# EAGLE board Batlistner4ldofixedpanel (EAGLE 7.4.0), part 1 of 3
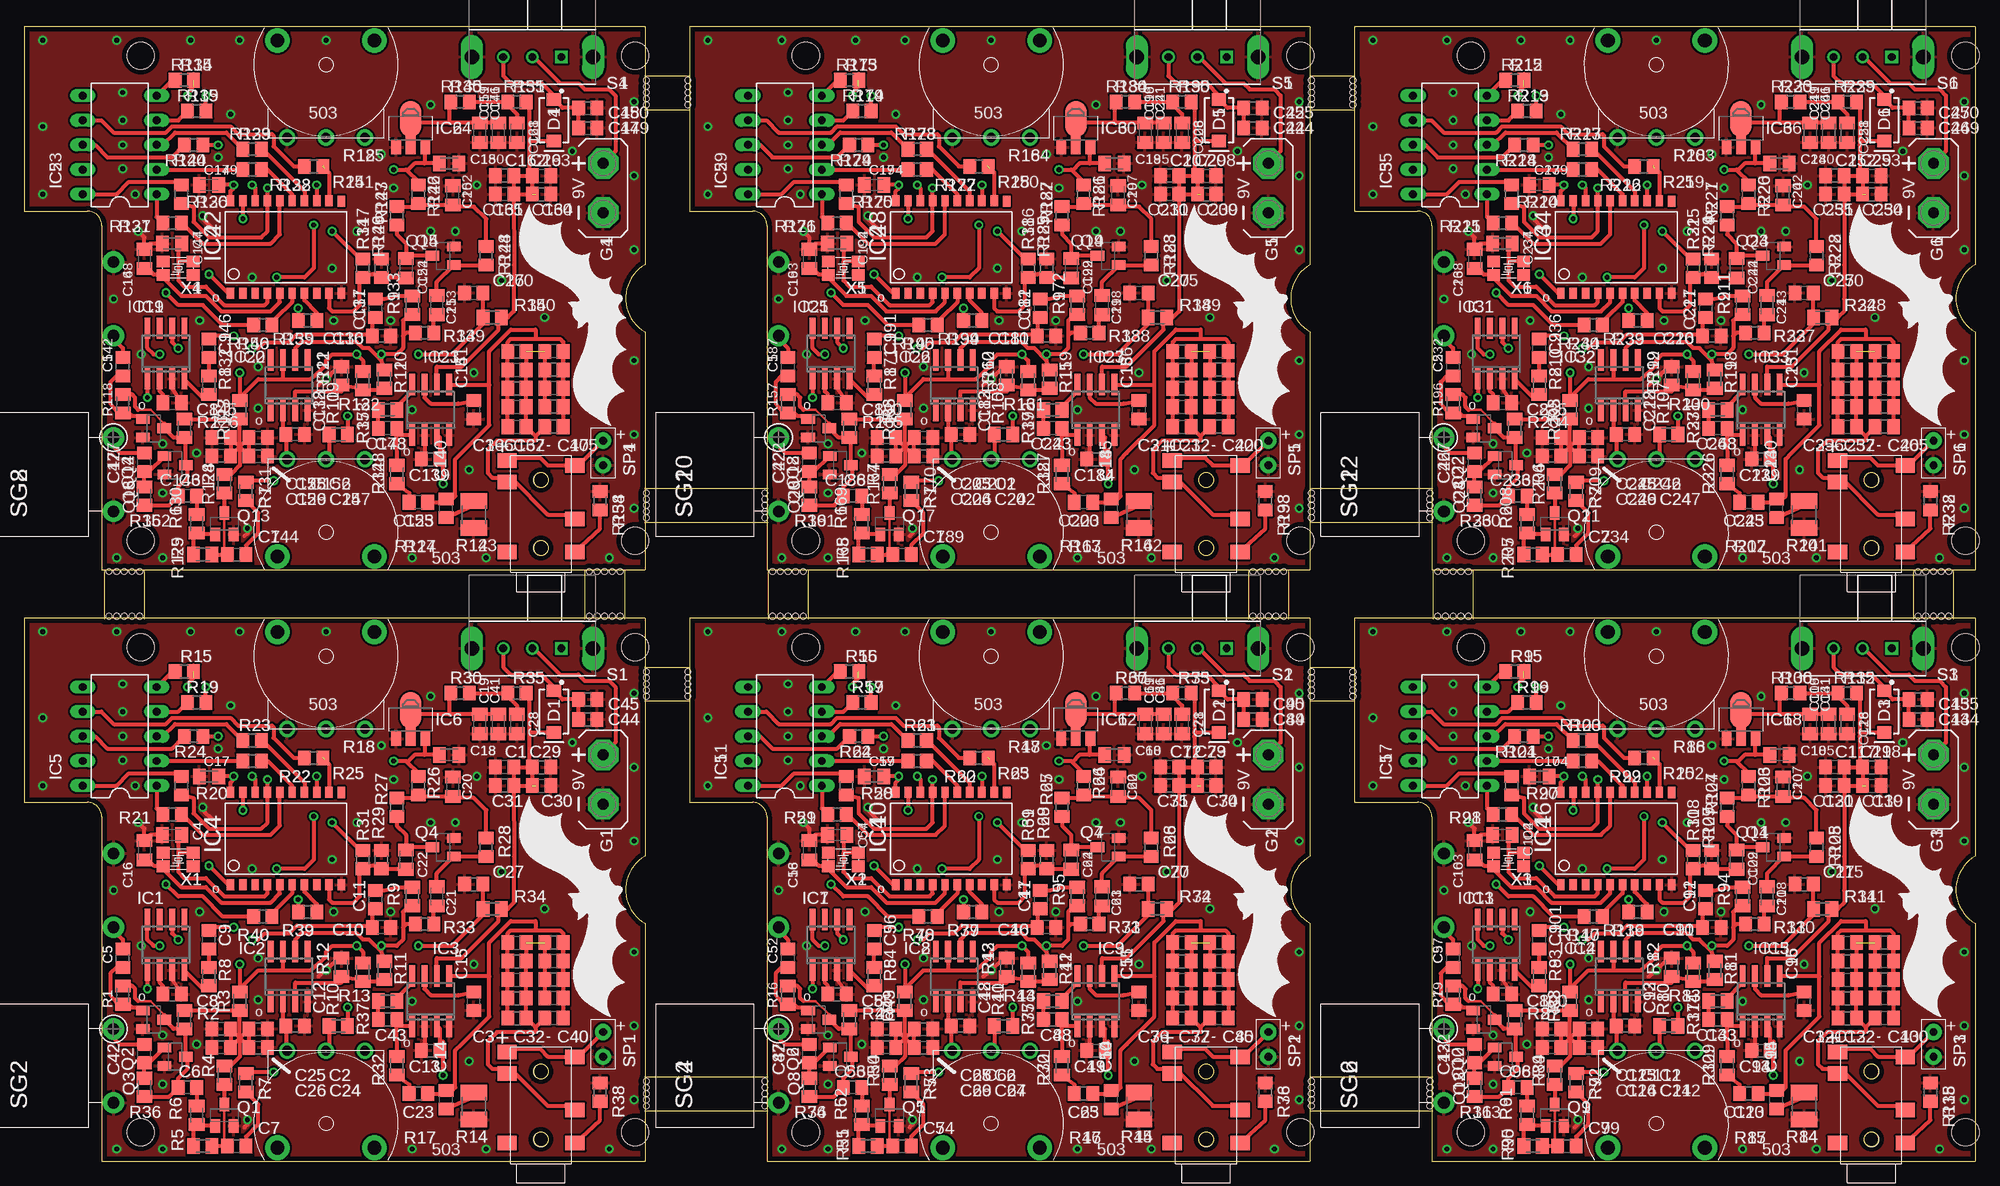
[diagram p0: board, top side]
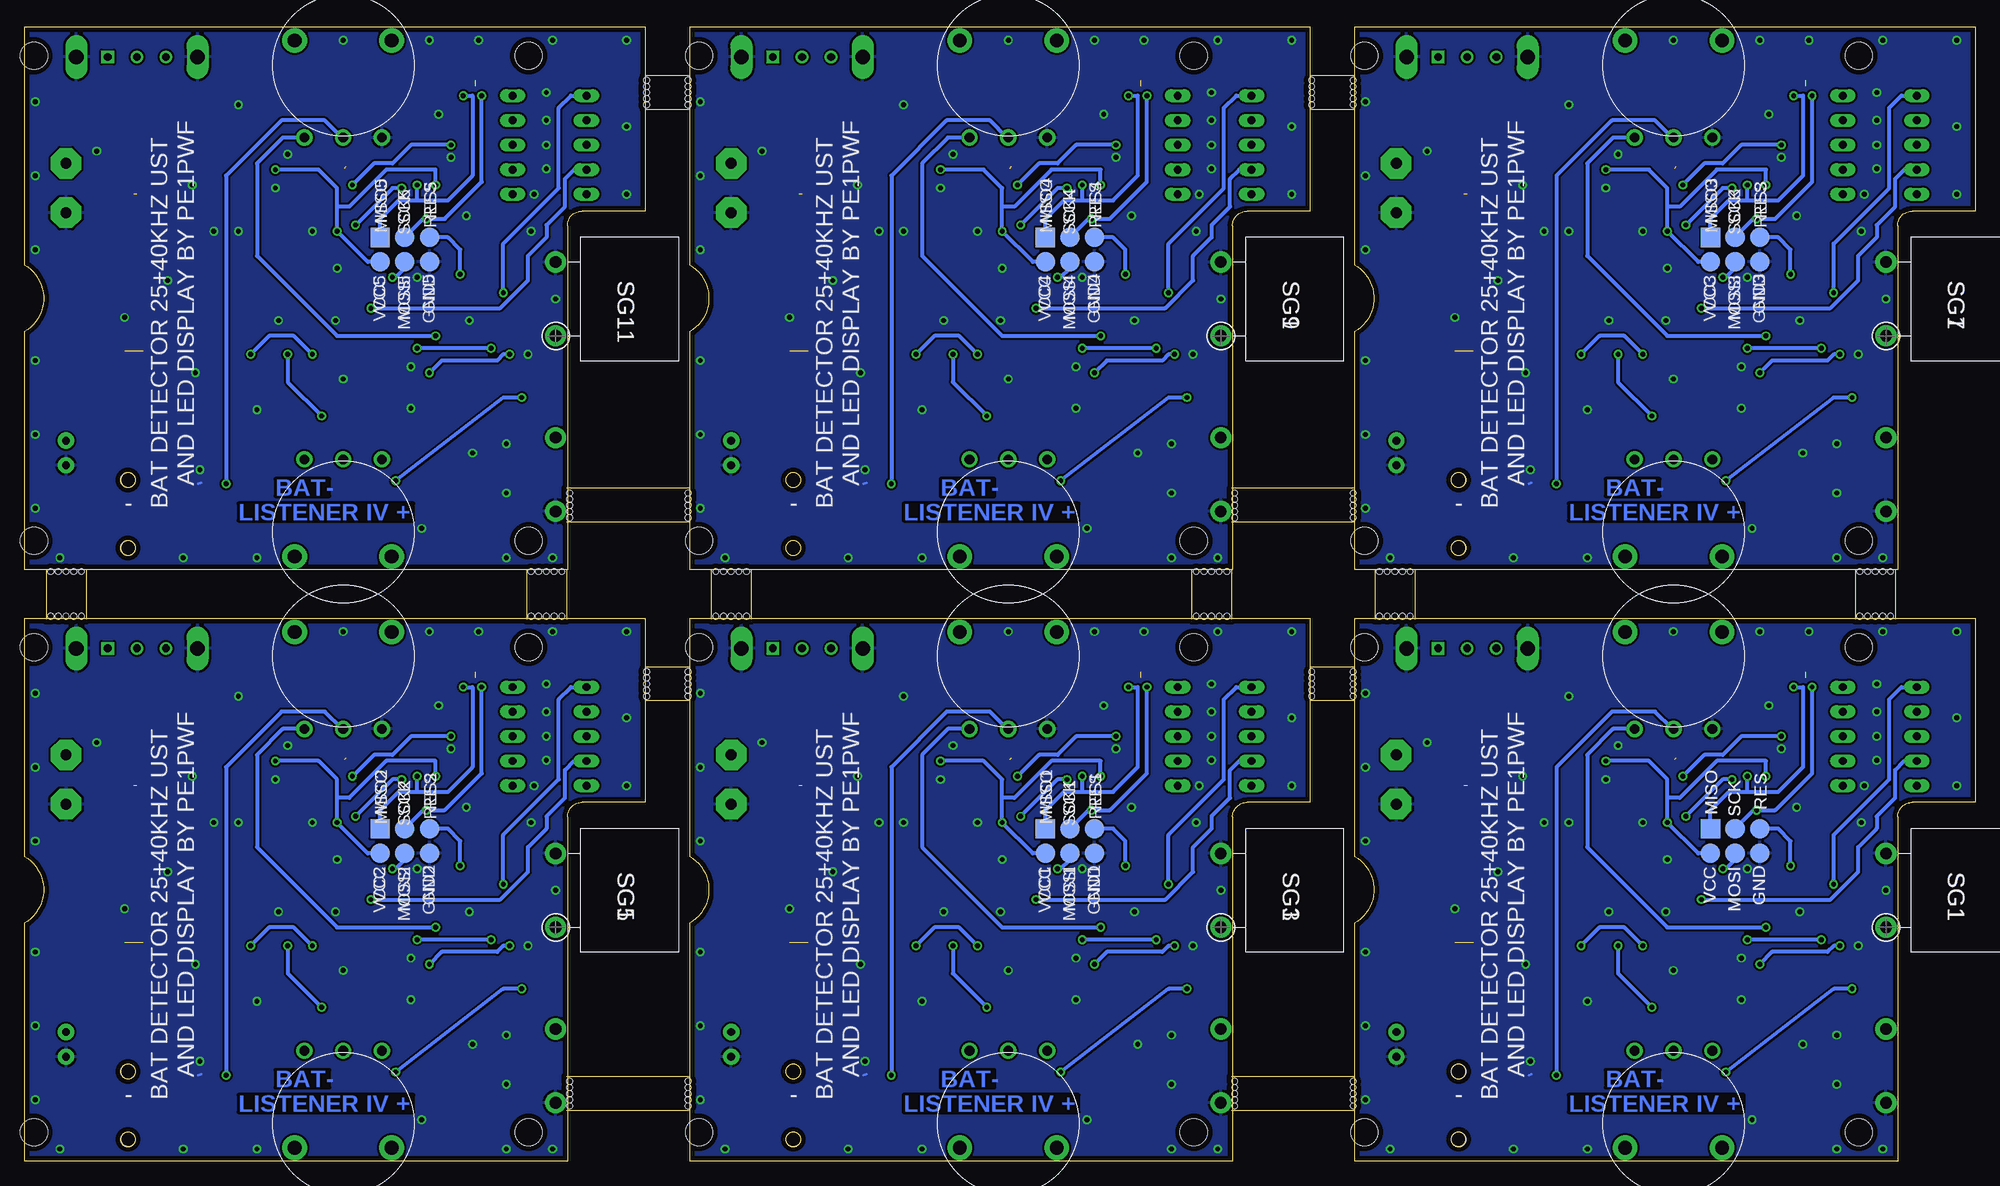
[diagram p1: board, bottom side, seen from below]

Size 201.16 x 116.96 mm. Coordinates in mm from the lower left corner, seen from the top.
Outline: 89 segments
Copper layers (1*16): Top 0.035mm / dielectric 1.5mm / Bottom 0.035mm
Design rules "default *": minimum track width 10mil, minimum drill 19mil, track to track 8mil, track to pad 8mil, pad to pad 8mil, via to via 8mil, smd to smd 8mil, copper to edge 20mil, drill to drill 8mil, minimum pad ring 10mil, minimum via ring 8mil, stop-mask expansion 4mil, vias tented up to drill 20mil, thermal gap 10mil
Holes 2.8 mm at 63,3 63,53 12,53 12,3 131.58,3 131.58,53 80.58,53 80.58,3 200.16,3 200.16,53 149.16,53 149.16,3 63,63.96 63,113.96 12,113.96 12,63.96 131.58,63.96 131.58,113.96 80.58,113.96 80.58,63.96 200.16,63.96 200.16,113.96 149.16,113.96 149.16,63.96
Holes 0.6 mm at 8.73,60.8 9.53,60.8 10.32,60.8 11.11,60.8 11.91,60.8 8.73,56.2 9.53,56.2 10.32,56.2 11.11,56.2 11.91,56.2 58.26,60.8 59.05,60.8 59.85,60.8 60.64,60.8 61.44,60.8 58.26,56.2 59.05,56.2 59.85,56.2 60.64,56.2 61.44,56.2 145.73,60.8 146.53,60.8 147.32,60.8 148.11,60.8 148.91,60.8 145.73,56.2 146.53,56.2 147.32,56.2 148.11,56.2 148.91,56.2 195.26,60.8 196.06,60.8 196.85,60.8 197.64,60.8 198.44,60.8 195.26,56.2 196.06,56.2 196.85,56.2 197.64,56.2 198.44,56.2 77.15,60.8 77.95,60.8 78.74,60.8 79.53,60.8 80.33,60.8 77.15,56.2 77.95,56.2 78.74,56.2 79.53,56.2 80.33,56.2 126.68,60.8 127.48,60.8 128.27,60.8 129.06,60.8 129.86,60.8 126.68,56.2 127.48,56.2 128.27,56.2 129.06,56.2 129.86,56.2 64.14,5.71 64.14,6.35 64.14,6.99 64.14,7.62 64.14,8.26 76.36,8.26 76.36,7.62 76.36,6.99 76.36,6.35 76.36,5.71 132.72,5.71 132.72,6.35 132.72,6.99 132.72,7.62 132.72,8.26 144.94,8.26 144.94,7.62 144.94,6.99 144.94,6.35 144.94,5.71 64.14,66.36 64.14,66.99 64.14,67.63 64.14,68.26 64.14,68.9 76.36,68.9 76.36,68.26 76.36,67.63 76.36,66.99 76.36,66.36 132.72,66.36 132.72,66.99 132.72,67.63 132.72,68.26 132.72,68.9 144.94,68.9 144.94,68.26 144.94,67.63 144.94,66.99 144.94,66.36 132.72,47.94 132.72,48.58 132.72,49.21 132.72,49.85 132.72,50.48 137,47.94 137,48.58 137,49.21 137,49.85 137,50.48 132.72,108.9 132.72,109.54 132.72,110.17 132.72,110.81 132.72,111.44 137,108.9 137,109.54 137,110.17 137,110.81 137,111.44 64.14,47.94 64.14,48.58 64.14,49.21 64.14,49.85 64.14,50.48 68.42,47.94 68.42,48.58 68.42,49.21 68.42,49.85 68.42,50.48 64.14,108.9 64.14,109.54 64.14,110.17 64.14,110.81 64.14,111.44 68.42,108.9 68.42,109.54 68.42,110.17 68.42,110.81 68.42,111.44

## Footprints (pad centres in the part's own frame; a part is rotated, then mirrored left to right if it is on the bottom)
C0805 = smd 1.3 x 1.5: 1 -0.95,0; 2 0.95,0
C0805K = smd 1.3 x 1.6: 1 -1,0; 2 1,0
SMA-DIODE = smd 1.27 x 1.47: A -2.15,0; C 2.15,0
AB9V = drill 1.118 pad 3.15 octagon: + 0,2.54; - 0,-2.54
TP20R = smd 2 x 2: TP 0,0
SO08 = smd 0.6 x 2.2: 1 -1.905,-2.6; 2 -0.635,-2.6; 3 0.635,-2.6; 4 1.905,-2.6; 5 1.905,2.6; 6 0.635,2.6; 7 -0.635,2.6; 8 -1.905,2.6
SO20L = smd 0.762 x 1.143: 1 -5.08,-5.131; 2 -3.81,-5.131; 3 -2.54,-5.131; 4 -1.27,-5.131; 5 0,-5.131; 6 1.27,-5.131; 7 2.54,-5.131; 8 3.81,-5.131; 9 5.08,-5.131; 10 6.35,-5.131; 11 6.35,4.369; 12 5.08,4.394; 13 3.81,4.394; 14 2.54,4.394; 15 1.27,4.394; 16 0,4.394; 17 -1.27,4.394; 18 -2.54,4.394; 19 -3.81,4.394; 20 -5.08,4.394
DIL10 = drill 0.813 long: 1 -5.08,-3.81; 2 -2.54,-3.81; 3 0,-3.81; 4 2.54,-3.81; 5 5.08,-3.81; 6 5.08,3.81; 7 2.54,3.81; 8 0,3.81; 9 -2.54,3.81; 10 -5.08,3.81
SOT89 = smd 1 x 1.5: 1 -1.499,-1.981; 3 1.499,-1.981 | smd 1 x 2: 2 0,-1.727 | smd 2.2 x 3.7: 2@1 0,0.94
TP20SQ = smd 2 x 2: TP 0,0
SOT23-BEC = smd 1 x 1.4: B -0.95,-1.1; C 0,1.1; E 0.95,-1.1
M0805 = smd 1.3 x 1.6: 1 -0.95,0; 2 0.95,0
R1210 = smd 1.6 x 2.7: 1 -1.4,0; 2 1.4,0
R0805 = smd 1.3 x 1.5: 1 -0.95,0; 2 0.95,0
RK10J11 = drill 1 pad 1.676: P$1 0,-7.5; P$2 -4,-7.5; P$3 4,-7.5 | drill 1.4 pad 2.54: P$4 5,2.5; P$5 -5,2.5
E-SWITCH_EG1206A_0 = drill 0.8 pad 1.3 square: 1 -3,3 | drill 0.8 pad 1.3: 2 0,3; 3 3,3 | drill 1.5 pad 1.778 long: 4 -6.25,3; 5 6.25,3
BMT1205XV7.5 = drill 1.2 pad 2.184: + 3.8,0; - -3.8,0
PADSONLY = drill 0.8 pad 1.676: + 0,0; - 0,-2.54
JW-PJ-342B = smd 1.5 x 2: P$1 4.1,1; P$2 4.1,8; P$3 7.5,1; P$4 11.3,8; P$5 13.5,8; P$6 13,1 | hole 1.5: 4.5,4.5; 11.5,4.5
IQG3225 = smd 1.3 x 1.2: 1 -1.55,-0.7; 2 1.55,-0.7; 3 1.55,0.7; 4 -1.55,0.7

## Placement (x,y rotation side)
C1  22uf  [C0805]  53.34,40.64 0 top
C2  22uf  [C0805]  24.13,13.65 0 top
C3  22uf  [C0805]  50.8,14.76 0 top
C4  22pF  [C0805K]  15.24,33.66 180 top
C5  1nF  [C0805]  10.16,20.95 90 top
C6  1nf  [C0805]  16.83,7.62 180 top
C7  1nF  [C0805]  21.91,1.59 0 top
C8  10nF  [C0805]  15.24,17.24 0 top
C9  47nF  [C0805]  19.05,22.86 90 top
C10  1nF  [C0805]  36.83,24.13 180 top
C11  47nF  [C0805]  36.2,26.99 270 top
C12  1.5nF  [C0805]  27.94,13.97 180 top
C13  10nF  [C0805]  41.91,11.43 0 top
C14  100nF  [C0805]  43.5,6.35 90 top
C15  10uF  [C0805]  46.35,16.51 90 top
C16  22pF  [C0805K]  12.38,32.07 90 top
C17  100nF  [C0805K]  19.05,39.69 0 top
C18  22uf  [C0805K]  43.81,41.91 0 top
C19  22uf  [C0805K]  46.99,45.09 270 top
C20  1uf  [C0805K]  44.2,38.61 90 top
C21  100nF  [C0805K]  42.55,27.3 90 top
C22  100nF  [C0805K]  39.37,31.11 270 top
C23  4.7nF  [C0805]  40.64,6.99 180 top
C24  22uf  [C0805]  24.13,11.75 0 top
C25  22uf  [C0805]  20.32,13.65 180 top
C26  22uf  [C0805]  20.32,11.75 180 top
C27  22uF  [C0805]  46.35,28.57 0 top
C28  22uf  [C0805K]  50.8,45.09 270 top
C29  22uf  [C0805]  53.34,38.73 0 top
C30  22uf  [C0805]  49.53,40.64 180 top
C31  22uf  [C0805]  49.53,38.73 180 top
C32  22uf  [C0805]  54.61,14.76 180 top
C33  22uf  [C0805]  54.61,16.83 180 top
C34  22uf  [C0805]  54.61,18.73 180 top
C35  22uf  [C0805]  54.61,20.64 180 top
C36  22uf  [C0805]  54.61,22.54 180 top
C37  22uf  [C0805]  50.8,22.54 0 top
C38  22uf  [C0805]  50.8,20.64 0 top
C39  22uf  [C0805]  50.8,18.73 0 top
C40  22uf  [C0805]  50.8,16.83 0 top
C41  22uf  [C0805K]  48.9,45.09 270 top
C42  1nF  [C0805]  12.38,11.11 90 top
C43  10uF  [C0805]  37.47,14.61 180 top
C44  22uf  [C0805]  58.1,45.56 0 top
C45  22uf  [C0805]  58.1,47.62 0 top
C46  1nF  [C0805]  105.41,24.13 180 top
C47  47nF  [C0805]  104.78,26.99 270 top
C48  1.5nF  [C0805]  96.52,13.97 180 top
C49  10nF  [C0805]  110.49,11.43 0 top
C50  100nF  [C0805]  112.08,6.35 90 top
C51  10uF  [C0805]  114.94,16.51 90 top
C52  1nF  [C0805]  78.74,20.95 90 top
C53  1nf  [C0805]  85.41,7.62 180 top
C54  1nF  [C0805]  90.49,1.59 0 top
C55  10nF  [C0805]  83.82,17.24 0 top
C56  47nF  [C0805]  87.63,22.86 90 top
C57  22pF  [C0805K]  83.82,33.66 180 top
C58  22pF  [C0805K]  80.96,32.07 90 top
C59  100nF  [C0805K]  87.63,39.69 0 top
C60  22uf  [C0805K]  112.39,41.91 0 top
C61  22uf  [C0805K]  115.57,45.09 270 top
C62  1uf  [C0805K]  112.78,38.61 90 top
C63  100nF  [C0805K]  111.12,27.3 90 top
C64  100nF  [C0805K]  107.95,31.11 270 top
C65  4.7nF  [C0805]  109.22,6.99 180 top
C66  22uf  [C0805]  92.71,13.65 0 top
C67  22uf  [C0805]  92.71,11.75 0 top
C68  22uf  [C0805]  88.9,13.65 180 top
C69  22uf  [C0805]  88.9,11.75 180 top
C70  22uF  [C0805]  114.94,28.57 0 top
C71  22uf  [C0805K]  119.38,45.09 270 top
C72  22uf  [C0805]  121.92,40.64 0 top
C73  22uf  [C0805]  121.92,38.73 0 top
C74  22uf  [C0805]  118.11,40.64 180 top
C75  22uf  [C0805]  118.11,38.73 180 top
C76  22uf  [C0805]  119.38,14.76 0 top
C77  22uf  [C0805]  123.19,14.76 180 top
C78  22uf  [C0805]  123.19,16.83 180 top
C79  22uf  [C0805]  123.19,18.73 180 top
C80  22uf  [C0805]  123.19,20.64 180 top
C81  22uf  [C0805]  123.19,22.54 180 top
C82  22uf  [C0805]  119.38,22.54 0 top
C83  22uf  [C0805]  119.38,20.64 0 top
C84  22uf  [C0805]  119.38,18.73 0 top
C85  22uf  [C0805]  119.38,16.83 0 top
C86  22uf  [C0805K]  117.47,45.09 270 top
C87  1nF  [C0805]  80.96,11.11 90 top
C88  10uF  [C0805]  106.05,14.61 180 top
C89  22uf  [C0805]  126.68,45.56 0 top
C90  22uf  [C0805]  126.68,47.62 0 top
C91  1nF  [C0805]  173.99,24.13 180 top
C92  47nF  [C0805]  173.35,26.99 270 top
C93  1.5nF  [C0805]  165.1,13.97 180 top
C94  10nF  [C0805]  179.07,11.43 0 top
C95  100nF  [C0805]  180.66,6.35 90 top
C96  10uF  [C0805]  183.51,16.51 90 top
C97  1nF  [C0805]  147.32,20.95 90 top
C98  1nf  [C0805]  153.99,7.62 180 top
C99  1nF  [C0805]  159.07,1.59 0 top
C100  10nF  [C0805]  152.4,17.24 0 top
C101  47nF  [C0805]  156.21,22.86 90 top
C102  22pF  [C0805K]  152.4,33.66 180 top
C103  22pF  [C0805K]  149.54,32.07 90 top
C104  100nF  [C0805K]  156.21,39.69 0 top
C105  22uf  [C0805K]  180.97,41.91 0 top
C106  22uf  [C0805K]  184.15,45.09 270 top
C107  1uf  [C0805K]  181.36,38.61 90 top
C108  100nF  [C0805K]  179.71,27.3 90 top
C109  100nF  [C0805K]  176.53,31.11 270 top
C110  4.7nF  [C0805]  177.8,6.99 180 top
C111  22uf  [C0805]  161.29,13.65 0 top
C112  22uf  [C0805]  161.29,11.75 0 top
C113  22uf  [C0805]  157.48,13.65 180 top
C114  22uf  [C0805]  157.48,11.75 180 top
C115  22uF  [C0805]  183.51,28.57 0 top
C116  22uf  [C0805K]  187.96,45.09 270 top
C117  22uf  [C0805]  190.5,40.64 0 top
C118  22uf  [C0805]  190.5,38.73 0 top
C119  22uf  [C0805]  186.69,40.64 180 top
C120  22uf  [C0805]  186.69,38.73 180 top
C121  22uf  [C0805]  187.96,14.76 0 top
C122  22uf  [C0805]  191.77,14.76 180 top
C123  22uf  [C0805]  191.77,16.83 180 top
C124  22uf  [C0805]  191.77,18.73 180 top
C125  22uf  [C0805]  191.77,20.64 180 top
C126  22uf  [C0805]  191.77,22.54 180 top
C127  22uf  [C0805]  187.96,22.54 0 top
C128  22uf  [C0805]  187.96,20.64 0 top
C129  22uf  [C0805]  187.96,18.73 0 top
C130  22uf  [C0805]  187.96,16.83 0 top
C131  22uf  [C0805K]  186.06,45.09 270 top
C132  1nF  [C0805]  149.54,11.11 90 top
C133  10uF  [C0805]  174.62,14.61 180 top
C134  22uf  [C0805]  195.26,45.56 0 top
C135  22uf  [C0805]  195.26,47.62 0 top
C136  1nF  [C0805]  36.83,85.09 180 top
C137  47nF  [C0805]  36.2,87.95 270 top
C138  1.5nF  [C0805]  27.94,74.93 180 top
C139  10nF  [C0805]  41.91,72.39 0 top
C140  100nF  [C0805]  43.5,67.31 90 top
C141  10uF  [C0805]  46.35,77.47 90 top
C142  1nF  [C0805]  10.16,81.92 90 top
C143  1nf  [C0805]  16.83,68.58 180 top
C144  1nF  [C0805]  21.91,62.55 0 top
C145  10nF  [C0805]  15.24,78.2 0 top
C146  47nF  [C0805]  19.05,83.82 90 top
C147  22pF  [C0805K]  15.24,94.61 180 top
C148  22pF  [C0805K]  12.38,93.03 90 top
C149  100nF  [C0805K]  19.05,100.65 0 top
C150  22uf  [C0805K]  43.81,102.87 0 top
C151  22uf  [C0805K]  46.99,106.05 270 top
C152  1uf  [C0805K]  44.2,99.57 90 top
C153  100nF  [C0805K]  42.55,88.27 90 top
C154  100nF  [C0805K]  39.37,92.08 270 top
C155  4.7nF  [C0805]  40.64,67.94 180 top
C156  22uf  [C0805]  24.13,74.61 0 top
C157  22uf  [C0805]  24.13,72.71 0 top
C158  22uf  [C0805]  20.32,74.61 180 top
C159  22uf  [C0805]  20.32,72.71 180 top
C160  22uF  [C0805]  46.35,89.53 0 top
C161  22uf  [C0805K]  50.8,106.05 270 top
C162  22uf  [C0805]  53.34,101.6 0 top
C163  22uf  [C0805]  53.34,99.69 0 top
C164  22uf  [C0805]  49.53,101.6 180 top
C165  22uf  [C0805]  49.53,99.69 180 top
C166  22uf  [C0805]  50.8,75.72 0 top
C167  22uf  [C0805]  54.61,75.72 180 top
C168  22uf  [C0805]  54.61,77.79 180 top
C169  22uf  [C0805]  54.61,79.69 180 top
C170  22uf  [C0805]  54.61,81.6 180 top
C171  22uf  [C0805]  54.61,83.5 180 top
C172  22uf  [C0805]  50.8,83.5 0 top
C173  22uf  [C0805]  50.8,81.6 0 top
C174  22uf  [C0805]  50.8,79.69 0 top
C175  22uf  [C0805]  50.8,77.79 0 top
C176  22uf  [C0805K]  48.9,106.05 270 top
C177  1nF  [C0805]  12.38,72.07 90 top
C178  10uF  [C0805]  37.47,75.56 180 top
C179  22uf  [C0805]  58.1,106.52 0 top
C180  22uf  [C0805]  58.1,108.58 0 top
C181  1nF  [C0805]  105.41,85.09 180 top
C182  47nF  [C0805]  104.78,87.95 270 top
C183  1.5nF  [C0805]  96.52,74.93 180 top
C184  10nF  [C0805]  110.49,72.39 0 top
C185  100nF  [C0805]  112.08,67.31 90 top
C186  10uF  [C0805]  114.94,77.47 90 top
C187  1nF  [C0805]  78.74,81.92 90 top
C188  1nf  [C0805]  85.41,68.58 180 top
C189  1nF  [C0805]  90.49,62.55 0 top
C190  10nF  [C0805]  83.82,78.2 0 top
C191  47nF  [C0805]  87.63,83.82 90 top
C192  22pF  [C0805K]  83.82,94.61 180 top
C193  22pF  [C0805K]  80.96,93.03 90 top
C194  100nF  [C0805K]  87.63,100.65 0 top
C195  22uf  [C0805K]  112.39,102.87 0 top
C196  22uf  [C0805K]  115.57,106.05 270 top
C197  1uf  [C0805K]  112.78,99.57 90 top
C198  100nF  [C0805K]  111.12,88.27 90 top
C199  100nF  [C0805K]  107.95,92.08 270 top
C200  4.7nF  [C0805]  109.22,67.94 180 top
C201  22uf  [C0805]  92.71,74.61 0 top
C202  22uf  [C0805]  92.71,72.71 0 top
C203  22uf  [C0805]  88.9,74.61 180 top
C204  22uf  [C0805]  88.9,72.71 180 top
C205  22uF  [C0805]  114.94,89.53 0 top
C206  22uf  [C0805K]  119.38,106.05 270 top
C207  22uf  [C0805]  121.92,101.6 0 top
C208  22uf  [C0805]  121.92,99.69 0 top
C209  22uf  [C0805]  118.11,101.6 180 top
C210  22uf  [C0805]  118.11,99.69 180 top
C211  22uf  [C0805]  119.38,75.72 0 top
C212  22uf  [C0805]  123.19,75.72 180 top
C213  22uf  [C0805]  123.19,77.79 180 top
C214  22uf  [C0805]  123.19,79.69 180 top
C215  22uf  [C0805]  123.19,81.6 180 top
C216  22uf  [C0805]  123.19,83.5 180 top
C217  22uf  [C0805]  119.38,83.5 0 top
C218  22uf  [C0805]  119.38,81.6 0 top
C219  22uf  [C0805]  119.38,79.69 0 top
C220  22uf  [C0805]  119.38,77.79 0 top
C221  22uf  [C0805K]  117.47,106.05 270 top
C222  1nF  [C0805]  80.96,72.07 90 top
C223  10uF  [C0805]  106.05,75.56 180 top
C224  22uf  [C0805]  126.68,106.52 0 top
C225  22uf  [C0805]  126.68,108.58 0 top
C226  1nF  [C0805]  173.99,85.09 180 top
C227  47nF  [C0805]  173.35,87.95 270 top
C228  1.5nF  [C0805]  165.1,74.93 180 top
C229  10nF  [C0805]  179.07,72.39 0 top
C230  100nF  [C0805]  180.66,67.31 90 top
C231  10uF  [C0805]  183.51,77.47 90 top
C232  1nF  [C0805]  147.32,81.92 90 top
C233  1nf  [C0805]  153.99,68.58 180 top
C234  1nF  [C0805]  159.07,62.55 0 top
C235  10nF  [C0805]  152.4,78.2 0 top
C236  47nF  [C0805]  156.21,83.82 90 top
C237  22pF  [C0805K]  152.4,94.61 180 top
C238  22pF  [C0805K]  149.54,93.03 90 top
C239  100nF  [C0805K]  156.21,100.65 0 top
C240  22uf  [C0805K]  180.97,102.87 0 top
C241  22uf  [C0805K]  184.15,106.05 270 top
C242  1uf  [C0805K]  181.36,99.57 90 top
C243  100nF  [C0805K]  179.71,88.27 90 top
C244  100nF  [C0805K]  176.53,92.08 270 top
C245  4.7nF  [C0805]  177.8,67.94 180 top
C246  22uf  [C0805]  161.29,74.61 0 top
C247  22uf  [C0805]  161.29,72.71 0 top
C248  22uf  [C0805]  157.48,74.61 180 top
C249  22uf  [C0805]  157.48,72.71 180 top
C250  22uF  [C0805]  183.51,89.53 0 top
C251  22uf  [C0805K]  187.96,106.05 270 top
C252  22uf  [C0805]  190.5,101.6 0 top
C253  22uf  [C0805]  190.5,99.69 0 top
C254  22uf  [C0805]  186.69,101.6 180 top
C255  22uf  [C0805]  186.69,99.69 180 top
C256  22uf  [C0805]  187.96,75.72 0 top
C257  22uf  [C0805]  191.77,75.72 180 top
C258  22uf  [C0805]  191.77,77.79 180 top
C259  22uf  [C0805]  191.77,79.69 180 top
C260  22uf  [C0805]  191.77,81.6 180 top
C261  22uf  [C0805]  191.77,83.5 180 top
C262  22uf  [C0805]  187.96,83.5 0 top
C263  22uf  [C0805]  187.96,81.6 0 top
C264  22uf  [C0805]  187.96,79.69 0 top
C265  22uf  [C0805]  187.96,77.79 0 top
C266  22uf  [C0805K]  186.06,106.05 270 top
C267  1nF  [C0805]  149.54,72.07 90 top
C268  10uF  [C0805]  174.62,75.56 180 top
C269  22uf  [C0805]  195.26,106.52 0 top
C270  22uf  [C0805]  195.26,108.58 0 top
D1  SS14  [SMA-DIODE]  54.61,46.35 270 top
D2  SS14  [SMA-DIODE]  123.19,46.35 270 top
D3  SS14  [SMA-DIODE]  191.77,46.35 270 top
D4  SS14  [SMA-DIODE]  54.61,107.31 270 top
D5  SS14  [SMA-DIODE]  123.19,107.31 270 top
D6  SS14  [SMA-DIODE]  191.77,107.31 270 top
G1  AB9V  [AB9V]  59.69,39.37 0 top
G2  AB9V  [AB9V]  128.27,39.37 0 top
G3  AB9V  [AB9V]  196.85,39.37 0 top
G4  AB9V  [AB9V]  59.69,100.33 0 top
G5  AB9V  [AB9V]  128.27,100.33 0 top
G6  AB9V  [AB9V]  196.85,100.33 0 top
GND  PTR1TP20R  [TP20R]  22.23,31.75 0 bottom
GND1  PTR1TP20R  [TP20R]  90.81,31.75 0 bottom
GND2  PTR1TP20R  [TP20R]  159.38,31.75 0 bottom
GND3  PTR1TP20R  [TP20R]  22.23,92.71 0 bottom
GND4  PTR1TP20R  [TP20R]  90.81,92.71 0 bottom
GND5  PTR1TP20R  [TP20R]  159.38,92.71 0 bottom
IC1  SA602  [SO08]  14.61,22.32 0 top
IC2  TL071D  [SO08]  27.3,19.05 0 top
IC3  LM386M-1  [SO08]  41.91,16.51 0 top
IC4  AT90S2313S  [SO20L]  26.35,33.66 0 top
IC5  [DIL10]  9.84,43.81 90 top
IC6  HT7550  [SOT89]  39.85,45.56 0 top
IC7  SA602  [SO08]  83.19,22.32 0 top
IC8  TL071D  [SO08]  95.89,19.05 0 top
IC9  LM386M-1  [SO08]  110.49,16.51 0 top
IC10  AT90S2313S  [SO20L]  94.93,33.66 0 top
IC11  [DIL10]  78.42,43.81 90 top
IC12  HT7550  [SOT89]  108.43,45.56 0 top
IC13  SA602  [SO08]  151.76,22.32 0 top
IC14  TL071D  [SO08]  164.47,19.05 0 top
IC15  LM386M-1  [SO08]  179.07,16.51 0 top
IC16  AT90S2313S  [SO20L]  163.51,33.66 0 top
IC17  [DIL10]  147,43.81 90 top
IC18  HT7550  [SOT89]  177.01,45.56 0 top
IC19  SA602  [SO08]  14.61,83.28 0 top
IC20  TL071D  [SO08]  27.3,80.01 0 top
IC21  LM386M-1  [SO08]  41.91,77.47 0 top
IC22  AT90S2313S  [SO20L]  26.35,94.61 0 top
IC23  [DIL10]  9.84,104.78 90 top
IC24  HT7550  [SOT89]  39.85,106.52 0 top
IC25  SA602  [SO08]  83.19,83.28 0 top
IC26  TL071D  [SO08]  95.89,80.01 0 top
IC27  LM386M-1  [SO08]  110.49,77.47 0 top
IC28  AT90S2313S  [SO20L]  94.93,94.61 0 top
IC29  [DIL10]  78.42,104.78 90 top
IC30  HT7550  [SOT89]  108.43,106.52 0 top
IC31  SA602  [SO08]  151.76,83.28 0 top
IC32  TL071D  [SO08]  164.47,80.01 0 top
IC33  LM386M-1  [SO08]  179.07,77.47 0 top
IC34  AT90S2313S  [SO20L]  163.51,94.61 0 top
IC35  [DIL10]  147,104.78 90 top
IC36  HT7550  [SOT89]  177.01,106.52 0 top
MISO  PTR1TP20SQ  [TP20SQ]  27.3,34.29 0 bottom
MISO1  PTR1TP20SQ  [TP20SQ]  95.89,34.29 0 bottom
MISO2  PTR1TP20SQ  [TP20SQ]  164.47,34.29 0 bottom
MISO3  PTR1TP20SQ  [TP20SQ]  27.3,95.25 0 bottom
MISO4  PTR1TP20SQ  [TP20SQ]  95.89,95.25 0 bottom
MISO5  PTR1TP20SQ  [TP20SQ]  164.47,95.25 0 bottom
MOSI  PTR1TP20R  [TP20R]  24.77,31.75 0 bottom
MOSI1  PTR1TP20R  [TP20R]  93.34,31.75 0 bottom
MOSI2  PTR1TP20R  [TP20R]  161.93,31.75 0 bottom
MOSI3  PTR1TP20R  [TP20R]  24.77,92.71 0 bottom
MOSI4  PTR1TP20R  [TP20R]  93.34,92.71 0 bottom
MOSI5  PTR1TP20R  [TP20R]  161.93,92.71 0 bottom
Q1  BC850SMD  [SOT23-BEC]  20.64,4.76 0 top
Q2  BC850SMD  [SOT23-BEC]  13.34,14.61 270 top
Q3  BC850SMD  [SOT23-BEC]  15.56,10.79 270 top
Q4  BC850SMD  [SOT23-BEC]  43.18,32.38 90 top
Q5  BC850SMD  [SOT23-BEC]  89.22,4.76 0 top
Q6  BC850SMD  [SOT23-BEC]  81.92,14.61 270 top
Q7  BC850SMD  [SOT23-BEC]  111.76,32.38 90 top
Q8  BC850SMD  [SOT23-BEC]  84.14,10.79 270 top
Q9  BC850SMD  [SOT23-BEC]  157.8,4.76 0 top
Q10  BC850SMD  [SOT23-BEC]  150.5,14.61 270 top
Q11  BC850SMD  [SOT23-BEC]  180.34,32.38 90 top
Q12  BC850SMD  [SOT23-BEC]  152.72,10.79 270 top
Q13  BC850SMD  [SOT23-BEC]  20.64,65.72 0 top
Q14  BC850SMD  [SOT23-BEC]  13.34,75.56 270 top
Q15  BC850SMD  [SOT23-BEC]  43.18,93.34 90 top
Q16  BC850SMD  [SOT23-BEC]  15.56,71.75 270 top
Q17  BC850SMD  [SOT23-BEC]  89.22,65.72 0 top
Q18  BC850SMD  [SOT23-BEC]  81.92,75.56 270 top
Q19  BC850SMD  [SOT23-BEC]  111.76,93.34 90 top
Q20  BC850SMD  [SOT23-BEC]  84.14,71.75 270 top
Q21  BC850SMD  [SOT23-BEC]  157.8,65.72 0 top
Q22  BC850SMD  [SOT23-BEC]  150.5,75.56 270 top
Q23  BC850SMD  [SOT23-BEC]  180.34,93.34 90 top
Q24  BC850SMD  [SOT23-BEC]  152.72,71.75 270 top
R1  220k  [M0805]  10.16,17.14 90 top
R2  4k7  [M0805]  16.51,14.61 270 top
R3  220r  [M0805]  22.23,16.51 270 top
R4  2k2  [M0805]  20.64,8.89 270 top
R5  220k  [M0805]  18.41,1.59 180 top
R6  10k  [M0805]  17.78,4.76 90 top
R7  100r  [M0805]  22.86,8.1 90 top
R8  4k7  [M0805]  19.05,19.05 90 top
R9  22k  [M0805]  40.01,27.3 90 top
R10  4k7  [M0805]  32.38,13.97 0 top
R11  470k  [M0805]  37.15,19.68 90 top
R12  220k  [M0805]  32.7,20 270 top
R13  220k  [M0805]  34.92,19.51 270 top
R14  10r  [R1210]  46.35,5.71 270 top
R15  2k2  [R0805]  16.51,50.48 180 top
R16  220k  [M0805]  78.74,17.14 90 top
R17  503  [RK10J11]  31.11,3.9 180 top
R18  503  [RK10J11]  31.11,52.07 0 top
R19  2k2  [R0805]  17.78,47.31 180 top
R20  2k2  [R0805]  16.19,38.73 90 top
R21  2k2  [R0805]  15.24,35.75 180 top
R22  2k2  [R0805]  23.5,41.27 180 top
R23  2k2  [R0805]  23.5,43.37 180 top
R24  2k2  [R0805]  17.46,43.81 180 top
R25  2k2  [R0805]  29.84,41.59 180 top
R26  100  [R0805]  40.64,38.73 270 top
R27  51k  [R0805]  38.42,36.51 270 top
R28  2M  [R0805]  47.62,32.38 270 top
R29  43k  [R0805]  34.92,31.11 270 top
R30  4.7  [R0805]  44.96,48.26 180 top
R31  33k  [R0805]  36.83,31.11 90 top
R32  2.2k  [M0805]  38.42,9.84 90 top
R33  10k  [R0805]  41.27,24.45 0 top
R34  10  [M0805]  48.26,26.04 0 top
R35  4.7  [R0805]  50.8,48.26 180 top
R36  220k  [M0805]  12.38,7.62 270 top
R37  1.2k  [M0805]  37.47,16.51 0 top
R38  100  [R0805]  59.37,7.14 270 top
R39  1k  [R0805]  29.21,25.72 180 top
R40  1k  [R0805]  24.61,25.24 180 top
R41  4k7  [M0805]  100.97,13.97 0 top
R42  470k  [M0805]  105.73,19.68 90 top
R43  220k  [M0805]  101.28,20 270 top
R44  220k  [M0805]  103.5,19.51 270 top
R45  10r  [R1210]  114.94,5.71 270 top
R46  503  [RK10J11]  99.69,3.9 180 top
R47  503  [RK10J11]  99.69,52.07 0 top
R48  4k7  [M0805]  85.09,14.61 270 top
R49  220r  [M0805]  90.81,16.51 270 top
R50  2k2  [M0805]  89.22,8.89 270 top
R51  220k  [M0805]  87,1.59 180 top
R52  10k  [M0805]  86.36,4.76 90 top
R53  100r  [M0805]  91.44,8.1 90 top
R54  4k7  [M0805]  87.63,19.05 90 top
R55  22k  [M0805]  108.58,27.3 90 top
R56  2k2  [R0805]  85.09,50.48 180 top
R57  2k2  [R0805]  86.36,47.31 180 top
R58  2k2  [R0805]  84.77,38.73 90 top
R59  2k2  [R0805]  83.82,35.75 180 top
R60  2k2  [R0805]  92.08,41.27 180 top
R61  2k2  [R0805]  92.08,43.37 180 top
R62  2k2  [R0805]  86.04,43.81 180 top
R63  2k2  [R0805]  98.42,41.59 180 top
R64  100  [R0805]  109.22,38.73 270 top
R65  51k  [R0805]  107,36.51 270 top
R66  2M  [R0805]  116.2,32.38 270 top
R67  4.7  [R0805]  113.54,48.26 180 top
R68  43k  [R0805]  103.5,31.11 270 top
R69  33k  [R0805]  105.41,31.11 90 top
R70  2.2k  [M0805]  107,9.84 90 top
R71  10k  [R0805]  109.86,24.45 0 top
R72  10  [M0805]  116.84,26.04 0 top
R73  4.7  [R0805]  119.38,48.26 180 top
R74  220k  [M0805]  80.96,7.62 270 top
R75  1.2k  [M0805]  106.05,16.51 0 top
R76  100  [R0805]  127.95,7.14 270 top
R77  1k  [R0805]  97.79,25.72 180 top
R78  1k  [R0805]  93.19,25.24 180 top
R79  220k  [M0805]  147.32,17.14 90 top
R80  4k7  [M0805]  169.54,13.97 0 top
R81  470k  [M0805]  174.31,19.68 90 top
R82  220k  [M0805]  169.86,20 270 top
R83  220k  [M0805]  172.09,19.51 270 top
R84  10r  [R1210]  183.51,5.71 270 top
R85  503  [RK10J11]  168.28,3.9 180 top
R86  503  [RK10J11]  168.28,52.07 0 top
R87  4k7  [M0805]  153.67,14.61 270 top
R88  220r  [M0805]  159.38,16.51 270 top
R89  2k2  [M0805]  157.8,8.89 270 top
R90  220k  [M0805]  155.57,1.59 180 top
R91  10k  [M0805]  154.94,4.76 90 top
R92  100r  [M0805]  160.02,8.1 90 top
R93  4k7  [M0805]  156.21,19.05 90 top
R94  22k  [M0805]  177.16,27.3 90 top
R95  2k2  [R0805]  153.67,50.48 180 top
R96  2k2  [R0805]  154.94,47.31 180 top
R97  2k2  [R0805]  153.35,38.73 90 top
R98  2k2  [R0805]  152.4,35.75 180 top
R99  2k2  [R0805]  160.66,41.27 180 top
R100  2k2  [R0805]  160.66,43.37 180 top
R101  2k2  [R0805]  154.62,43.81 180 top
R102  2k2  [R0805]  167,41.59 180 top
R103  100  [R0805]  177.8,38.73 270 top
R104  51k  [R0805]  175.58,36.51 270 top
R105  2M  [R0805]  184.78,32.38 270 top
R106  4.7  [R0805]  182.12,48.26 180 top
R107  43k  [R0805]  172.09,31.11 270 top
R108  33k  [R0805]  173.99,31.11 90 top
R109  2.2k  [M0805]  175.58,9.84 90 top
R110  10k  [R0805]  178.44,24.45 0 top
R111  10  [M0805]  185.42,26.04 0 top
R112  4.7  [R0805]  187.96,48.26 180 top
R113  220k  [M0805]  149.54,7.62 270 top
R114  1.2k  [M0805]  174.62,16.51 0 top
R115  100  [R0805]  196.53,7.14 270 top
R116  1k  [R0805]  166.37,25.72 180 top
R117  1k  [R0805]  161.77,25.24 180 top
R118  220k  [M0805]  10.16,78.11 90 top
R119  4k7  [M0805]  32.38,74.93 0 top
R120  470k  [M0805]  37.15,80.64 90 top
R121  220k  [M0805]  32.7,80.96 270 top
R122  220k  [M0805]  34.92,80.47 270 top
R123  10r  [R1210]  46.35,66.67 270 top
R124  503  [RK10J11]  31.11,64.86 180 top
R125  503  [RK10J11]  31.11,113.03 0 top
R126  4k7  [M0805]  16.51,75.56 270 top
R127  220r  [M0805]  22.23,77.47 270 top
R128  2k2  [M0805]  20.64,69.85 270 top
R129  220k  [M0805]  18.41,62.55 180 top
R130  10k  [M0805]  17.78,65.72 90 top
R131  100r  [M0805]  22.86,69.06 90 top
R132  4k7  [M0805]  19.05,80.01 90 top
R133  22k  [M0805]  40.01,88.27 90 top
R134  2k2  [R0805]  16.51,111.44 180 top
R135  2k2  [R0805]  17.78,108.27 180 top
R136  2k2  [R0805]  16.19,99.69 90 top
R137  2k2  [R0805]  15.24,96.71 180 top
R138  2k2  [R0805]  23.5,102.23 180 top
R139  2k2  [R0805]  23.5,104.33 180 top
R140  2k2  [R0805]  17.46,104.78 180 top
R141  2k2  [R0805]  29.84,102.55 180 top
R142  100  [R0805]  40.64,99.69 270 top
R143  51k  [R0805]  38.42,97.47 270 top
R144  2M  [R0805]  47.62,93.34 270 top
R145  4.7  [R0805]  44.96,109.22 180 top
R146  43k  [R0805]  34.92,92.08 270 top
R147  33k  [R0805]  36.83,92.08 90 top
R148  2.2k  [M0805]  38.42,70.8 90 top
R149  10k  [R0805]  41.27,85.41 0 top
R150  10  [M0805]  48.26,87 0 top
R151  4.7  [R0805]  50.8,109.22 180 top
R152  220k  [M0805]  12.38,68.58 270 top
R153  1.2k  [M0805]  37.47,77.47 0 top
R154  100  [R0805]  59.37,68.1 270 top
R155  1k  [R0805]  29.21,86.68 180 top
R156  1k  [R0805]  24.61,86.2 180 top
R157  220k  [M0805]  78.74,78.11 90 top
R158  4k7  [M0805]  100.97,74.93 0 top
R159  470k  [M0805]  105.73,80.64 90 top
R160  220k  [M0805]  101.28,80.96 270 top
R161  220k  [M0805]  103.5,80.47 270 top
R162  10r  [R1210]  114.94,66.67 270 top
R163  503  [RK10J11]  99.69,64.86 180 top
R164  503  [RK10J11]  99.69,113.03 0 top
R165  4k7  [M0805]  85.09,75.56 270 top
R166  220r  [M0805]  90.81,77.47 270 top
R167  2k2  [M0805]  89.22,69.85 270 top
R168  220k  [M0805]  87,62.55 180 top
R169  10k  [M0805]  86.36,65.72 90 top
R170  100r  [M0805]  91.44,69.06 90 top
R171  4k7  [M0805]  87.63,80.01 90 top
R172  22k  [M0805]  108.58,88.27 90 top
R173  2k2  [R0805]  85.09,111.44 180 top
R174  2k2  [R0805]  86.36,108.27 180 top
R175  2k2  [R0805]  84.77,99.69 90 top
R176  2k2  [R0805]  83.82,96.71 180 top
R177  2k2  [R0805]  92.08,102.23 180 top
R178  2k2  [R0805]  92.08,104.33 180 top
R179  2k2  [R0805]  86.04,104.78 180 top
R180  2k2  [R0805]  98.42,102.55 180 top
R181  100  [R0805]  109.22,99.69 270 top
R182  51k  [R0805]  107,97.47 270 top
R183  2M  [R0805]  116.2,93.34 270 top
R184  4.7  [R0805]  113.54,109.22 180 top
R185  43k  [R0805]  103.5,92.08 270 top
R186  33k  [R0805]  105.41,92.08 90 top
R187  2.2k  [M0805]  107,70.8 90 top
R188  10k  [R0805]  109.86,85.41 0 top
R189  10  [M0805]  116.84,87 0 top
R190  4.7  [R0805]  119.38,109.22 180 top
R191  220k  [M0805]  80.96,68.58 270 top
R192  1.2k  [M0805]  106.05,77.47 0 top
R193  100  [R0805]  127.95,68.1 270 top
R194  1k  [R0805]  97.79,86.68 180 top
R195  1k  [R0805]  93.19,86.2 180 top
R196  220k  [M0805]  147.32,78.11 90 top
R197  4k7  [M0805]  169.54,74.93 0 top
R198  470k  [M0805]  174.31,80.64 90 top
R199  220k  [M0805]  169.86,80.96 270 top
R200  220k  [M0805]  172.09,80.47 270 top
R201  10r  [R1210]  183.51,66.67 270 top
R202  503  [RK10J11]  168.28,64.86 180 top
R203  503  [RK10J11]  168.28,113.03 0 top
R204  4k7  [M0805]  153.67,75.56 270 top
R205  220r  [M0805]  159.38,77.47 270 top
R206  2k2  [M0805]  157.8,69.85 270 top
R207  220k  [M0805]  155.57,62.55 180 top
R208  10k  [M0805]  154.94,65.72 90 top
R209  100r  [M0805]  160.02,69.06 90 top
R210  4k7  [M0805]  156.21,80.01 90 top
R211  22k  [M0805]  177.16,88.27 90 top
R212  2k2  [R0805]  153.67,111.44 180 top
R213  2k2  [R0805]  154.94,108.27 180 top
R214  2k2  [R0805]  153.35,99.69 90 top
R215  2k2  [R0805]  152.4,96.71 180 top
R216  2k2  [R0805]  160.66,102.23 180 top
R217  2k2  [R0805]  160.66,104.33 180 top
R218  2k2  [R0805]  154.62,104.78 180 top
R219  2k2  [R0805]  167,102.55 180 top
R220  100  [R0805]  177.8,99.69 270 top
R221  51k  [R0805]  175.58,97.47 270 top
R222  2M  [R0805]  184.78,93.34 270 top
R223  4.7  [R0805]  182.12,109.22 180 top
R224  43k  [R0805]  172.09,92.08 270 top
R225  33k  [R0805]  173.99,92.08 90 top
R226  2.2k  [M0805]  175.58,70.8 90 top
R227  10k  [R0805]  178.44,85.41 0 top
R228  10  [M0805]  185.42,87 0 top
R229  4.7  [R0805]  187.96,109.22 180 top
R230  220k  [M0805]  149.54,68.58 270 top
R231  1.2k  [M0805]  174.62,77.47 0 top
R232  100  [R0805]  196.53,68.1 270 top
R233  1k  [R0805]  166.37,86.68 180 top
R234  1k  [R0805]  161.77,86.2 180 top
RES  PTR1TP20R  [TP20R]  22.23,34.29 0 bottom
RES1  PTR1TP20R  [TP20R]  90.81,34.29 0 bottom
RES2  PTR1TP20R  [TP20R]  159.38,34.29 0 bottom
RES3  PTR1TP20R  [TP20R]  22.23,95.25 0 bottom
RES4  PTR1TP20R  [TP20R]  90.81,95.25 0 bottom
RES5  PTR1TP20R  [TP20R]  159.38,95.25 0 bottom
S1  E-SWITCH_EG1206AE-SWITCH_EG1206A_0_0  [E-SWITCH_EG1206A_0]  52.39,55.88 180 top
S2  E-SWITCH_EG1206AE-SWITCH_EG1206A_0_0  [E-SWITCH_EG1206A_0]  120.97,55.88 180 top
S3  E-SWITCH_EG1206AE-SWITCH_EG1206A_0_0  [E-SWITCH_EG1206A_0]  189.55,55.88 180 top
S4  E-SWITCH_EG1206AE-SWITCH_EG1206A_0_0  [E-SWITCH_EG1206A_0]  52.39,116.84 180 top
S5  E-SWITCH_EG1206AE-SWITCH_EG1206A_0_0  [E-SWITCH_EG1206A_0]  120.97,116.84 180 top
S6  E-SWITCH_EG1206AE-SWITCH_EG1206A_0_0  [E-SWITCH_EG1206A_0]  189.55,116.84 180 top
SCK  PTR1TP20R  [TP20R]  24.77,34.29 0 bottom
SCK1  PTR1TP20R  [TP20R]  93.34,34.29 0 bottom
SCK2  PTR1TP20R  [TP20R]  161.93,34.29 0 bottom
SCK3  PTR1TP20R  [TP20R]  24.77,95.25 0 bottom
SCK4  PTR1TP20R  [TP20R]  93.34,95.25 0 bottom
SCK5  PTR1TP20R  [TP20R]  161.93,95.25 0 bottom
SG1  BMT1205XV7.5  [BMT1205XV7.5]  9.21,27.94 270 bottom
SG2  BMT1205XV7.5  [BMT1205XV7.5]  9.21,9.84 90 top
SG3  BMT1205XV7.5  [BMT1205XV7.5]  77.79,27.94 270 bottom
SG4  BMT1205XV7.5  [BMT1205XV7.5]  77.79,9.84 90 top
SG5  BMT1205XV7.5  [BMT1205XV7.5]  146.37,27.94 270 bottom
SG6  BMT1205XV7.5  [BMT1205XV7.5]  146.37,9.84 90 top
SG7  BMT1205XV7.5  [BMT1205XV7.5]  9.21,88.9 270 bottom
SG8  BMT1205XV7.5  [BMT1205XV7.5]  9.21,70.8 90 top
SG9  BMT1205XV7.5  [BMT1205XV7.5]  77.79,88.9 270 bottom
SG10  BMT1205XV7.5  [BMT1205XV7.5]  77.79,70.8 90 top
SG11  BMT1205XV7.5  [BMT1205XV7.5]  146.37,88.9 270 bottom
SG12  BMT1205XV7.5  [BMT1205XV7.5]  146.37,70.8 90 top
SP1  [PADSONLY]  59.69,13.34 0 top
SP2  [PADSONLY]  128.27,13.34 0 top
SP3  [PADSONLY]  196.85,13.34 0 top
SP4  [PADSONLY]  59.69,74.3 0 top
SP5  [PADSONLY]  128.27,74.3 0 top
SP6  [PADSONLY]  196.85,74.3 0 top
U$1  JW-PJ-342B  [JW-PJ-342B]  57.78,-2.22 90 top
U$2  JW-PJ-342B  [JW-PJ-342B]  126.36,-2.22 90 top
U$3  JW-PJ-342B  [JW-PJ-342B]  194.94,-2.22 90 top
U$4  JW-PJ-342B  [JW-PJ-342B]  57.78,58.74 90 top
U$5  JW-PJ-342B  [JW-PJ-342B]  126.36,58.74 90 top
U$6  JW-PJ-342B  [JW-PJ-342B]  194.94,58.74 90 top
VCC  PTR1TP20R  [TP20R]  27.3,31.75 0 bottom
VCC1  PTR1TP20R  [TP20R]  95.89,31.75 0 bottom
VCC2  PTR1TP20R  [TP20R]  164.47,31.75 0 bottom
VCC3  PTR1TP20R  [TP20R]  27.3,92.71 0 bottom
VCC4  PTR1TP20R  [TP20R]  95.89,92.71 0 bottom
VCC5  PTR1TP20R  [TP20R]  164.47,92.71 0 bottom
X1  SMCE-3225  [IQG3225]  15.88,31.11 180 top
X2  SMCE-3225  [IQG3225]  84.45,31.11 180 top
X3  SMCE-3225  [IQG3225]  153.03,31.11 180 top
X4  SMCE-3225  [IQG3225]  15.88,92.08 180 top
X5  SMCE-3225  [IQG3225]  84.45,92.08 180 top
X6  SMCE-3225  [IQG3225]  153.03,92.08 180 top

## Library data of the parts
C1-C270 R1-R16 R19-R45 R48-R84 R87-R123 R126-R162 R165-R201 R204-R234 = rcl
D1-D6 = SparkFun-DiscreteSemi; PROD_ID: DIO-08053; VALUE: 1A/40V/500mV
G1-G6 = battery
GND GND1-GND5 MISO MISO1-MISO5 MOSI MOSI1-MOSI5 RES RES1-RES5 SCK SCK1-SCK5 VCC VCC1-VCC5 = testpad
IC1-IC3 IC6-IC9 IC12-IC15 IC18-IC21 IC24-IC27 IC30-IC33 IC36 = linear
IC4 IC10 IC16 IC22 IC28 IC34 = atmel; OC_FARNELL: unknown; OC_NEWARK: unknown
IC5 IC11 IC17 IC23 IC29 IC35 = ic-package
Q1-Q24 = transistor-npn
R17 R18 R46 R47 R85 R86 R124 R125 R163 R164 R202 R203 = pe1pwf
S1-S6 = E-Switch - EG1206A; CENTROID_NOT_SPECIFIED: No; DATASHEET: http://spec_sheets.e-switch.com/specs/P040021.pdf; DIGIKEY_DESCRIPTION: SWITCH Slide Switch SPDT Through Hole, Right Angle; DIGIKEY_PART_NUMBER: EG1917-ND; LEAD_FREE: yes; MF: E-Switch; MOUSER_PART_NUMBER: 612-EG1206A; MPN: EG1206A; PACKAGE: SIP; PREFIX: SW; ROHS: yes; TEMPERATURE_RANGE_HIGH: +70°C; TEMPERATURE_RANGE_LOW: -20°C
SG1-SG12 SP1-SP6 = buzzer
U$1-U$6 = jack
X1-X6 = interquip

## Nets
+9V: C1.1 C29.1 C30.1 C31.1 D1.C IC3.6 R34.2 R35.1
+9V1: C72.1 C73.1 C74.1 C75.1 D2.C IC9.6 R72.2 R73.1
+9V2: C117.1 C118.1 C119.1 C120.1 D3.C IC15.6 R111.2 R112.1
+9V3: C162.1 C163.1 C164.1 C165.1 D4.C IC21.6 R150.2 R151.1
+9V4: C207.1 C208.1 C209.1 C210.1 D5.C IC27.6 R189.2 R190.1
+9V5: C252.1 C253.1 C254.1 C255.1 D6.C IC33.6 R228.2 R229.1
-1V: IC2.6 R9.1 R10.2 R11.2 R33.1
-1V1: IC8.6 R41.2 R42.2 R55.1 R71.1
-1V2: IC14.6 R80.2 R81.2 R94.1 R110.1
-1V3: IC20.6 R119.2 R120.2 R133.1 R149.1
-1V4: IC26.6 R158.2 R159.2 R172.1 R188.1
-1V5: IC32.6 R197.2 R198.2 R211.1 R227.1
GND: C1.2 C2.2 C4.2 C8.2 C10.1 C12.1 C13.1 C15.1 C16.2 C17.1 C18.2 C19.2 C20.2 C24.2 C25.2 C26.2 C27.1 C28.2 C29.2 C30.2 C31.2 C41.2 C44.2 C45.2 G1.- GND.TP IC1.3 IC2.4 IC3.2 IC3.4 IC4.10 IC6.1 Q1.E Q2.E Q3.E Q4.E R12.1 R14.2 R18.P$2 R31.2 R38.1 S1.4 S1.5 SG1.- SG2.- SP1.-
GND1: C46.1 C48.1 C49.1 C51.1 C55.2 C57.2 C58.2 C59.1 C60.2 C61.2 C62.2 C66.2 C67.2 C68.2 C69.2 C70.1 C71.2 C72.2 C73.2 C74.2 C75.2 C86.2 C89.2 C90.2 G2.- GND1.TP IC7.3 IC8.4 IC9.2 IC9.4 IC10.10 IC12.1 Q5.E Q6.E Q7.E Q8.E R43.1 R45.2 R47.P$2 R69.2 R76.1 S2.4 S2.5 SG3.- SG4.- SP2.-
GND2: C91.1 C93.1 C94.1 C96.1 C100.2 C102.2 C103.2 C104.1 C105.2 C106.2 C107.2 C111.2 C112.2 C113.2 C114.2 C115.1 C116.2 C117.2 C118.2 C119.2 C120.2 C131.2 C134.2 C135.2 G3.- GND2.TP IC13.3 IC14.4 IC15.2 IC15.4 IC16.10 IC18.1 Q9.E Q10.E Q11.E Q12.E R82.1 R84.2 R86.P$2 R108.2 R115.1 S3.4 S3.5 SG5.- SG6.- SP3.-
GND3: C136.1 C138.1 C139.1 C141.1 C145.2 C147.2 C148.2 C149.1 C150.2 C151.2 C152.2 C156.2 C157.2 C158.2 C159.2 C160.1 C161.2 C162.2 C163.2 C164.2 C165.2 C176.2 C179.2 C180.2 G4.- GND3.TP IC19.3 IC20.4 IC21.2 IC21.4 IC22.10 IC24.1 Q13.E Q14.E Q15.E Q16.E R121.1 R123.2 R125.P$2 R147.2 R154.1 S4.4 S4.5 SG7.- SG8.- SP4.-
GND4: C181.1 C183.1 C184.1 C186.1 C190.2 C192.2 C193.2 C194.1 C195.2 C196.2 C197.2 C201.2 C202.2 C203.2 C204.2 C205.1 C206.2 C207.2 C208.2 C209.2 C210.2 C221.2 C224.2 C225.2 G5.- GND4.TP IC25.3 IC26.4 IC27.2 IC27.4 IC28.10 IC30.1 Q17.E Q18.E Q19.E Q20.E R160.1 R162.2 R164.P$2 R186.2 R193.1 S5.4 S5.5 SG9.- SG10.- SP5.-
GND5: C226.1 C228.1 C229.1 C231.1 C235.2 C237.2 C238.2 C239.1 C240.2 C241.2 C242.2 C246.2 C247.2 C248.2 C249.2 C250.1 C251.2 C252.2 C253.2 C254.2 C255.2 C266.2 C269.2 C270.2 G6.- GND5.TP IC31.3 IC32.4 IC33.2 IC33.4 IC34.10 IC36.1 Q21.E Q22.E Q23.E Q24.E R199.1 R201.2 R203.P$2 R225.2 R232.1 S6.4 S6.5 SG11.- SG12.- SP6.-
N$1: C3.2 C32.2 C33.2 C34.2 C35.2 C36.2 C37.2 C38.2 C39.2 C40.2 U$1.P$3 U$1.P$4
N$2: C14.1 R14.1
N$3: C7.1 Q1.C R4.2 R5.1
N$4: C15.2 IC3.7
N$5: IC1.4 R8.1
N$6: C9.1 R8.2
N$7: C76.2 C77.2 C78.2 C79.2 C80.2 C81.2 C82.2 C83.2 C84.2 C85.2 U$2.P$3 U$2.P$4
N$8: IC2.3 R11.1 R12.2 R13.2
N$9: C44.1 C45.1 D1.A S1.3
N$10: C5.2 SG1.+
N$11: C5.1 Q2.B R1.1
N$12: C6.2 Q2.C Q3.C R1.2 R2.2 R36.2
N$13: C2.1 C24.1 C25.1 C26.1 R2.1 R3.2 R4.1
N$14: C7.2 R7.1
N$15: R10.1 R17.P$1
N$16: Q1.B R5.2 R6.1
N$17: C6.1 R6.2
N$18: IC1.1 R7.2
N$19: C8.1 IC1.2
N$20: C9.2 R18.P$3
N$21: C50.1 R45.1
N$22: C13.2 IC3.3 R18.P$1
N$23: C22.2 IC4.9 R29.2 R31.1
N$24: IC4.19 R15.1 SCK.TP
N$25: IC4.18 MISO.TP R19.1
N$26: IC4.17 MOSI.TP R20.1
N$27: C3.1 C14.2 C23.1 C32.1 C33.1 C34.1 C35.1 C36.1 C37.1 C38.1 C39.1 C40.1 IC3.5
N$28: C12.2 IC2.2 R17.P$3
N$29: IC4.16 R21.1
N$30: C10.2 C11.2 IC1.6
N$31: IC4.15 R22.1
N$32: C11.1 R9.2
N$33: IC4.14 R23.1
N$34: IC4.13 R24.1
N$35: IC4.12 R25.1
N$36: IC5.5 R15.2
N$37: IC5.4 R19.2
N$38: IC5.10 R20.2
N$39: IC5.1 R21.2
N$40: IC5.2 R22.2
N$41: IC5.3 R23.2
N$42: IC5.8 R24.2
N$43: IC5.7 R25.2
N$44: IC5.9 R39.2
N$45: IC5.6 R40.2
N$46: IC4.6 R40.1
N$47: C16.1 IC4.5 X1.3
N$48: C21.1 R33.2
N$49: C17.2 C18.1 IC4.20 IC6.3 R26.1 R29.1 VCC.TP
N$50: C23.2 R32.1
N$51: C20.1 R26.2 R27.1 R28.1
N$52: C21.2 Q4.B R28.2
N$53: C22.1 Q4.C R27.2
N$54: IC4.1 RES.TP
N$55: C19.1 C41.1 IC6.2@1 R30.2
N$56: C43.1 IC3.1 R32.2
N$57: C28.1 R30.1 R35.2
N$58: C42.2 SG2.+
N$59: C27.2 IC1.8 IC2.7 R3.1 R13.1 R34.1
N$60: C42.1 Q3.B R36.1
N$61: C43.2 R37.1
N$62: IC3.8 R37.2
N$63: C4.1 IC4.4 X1.1
N$64: R38.2 U$1.P$1
N$65: SP1.+ U$1.P$5 U$1.P$6
N$66: IC4.7 R39.1
N$67: G1.+ S1.2
N$68: C51.2 IC9.7
N$69: IC7.4 R54.1
N$70: C56.1 R54.2
N$71: C52.2 SG3.+
N$72: C52.1 Q6.B R16.1
N$73: C53.2 Q6.C Q8.C R16.2 R48.2 R74.2
N$74: C66.1 C67.1 C68.1 C69.1 R48.1 R49.2 R50.1
N$75: Q5.B R51.2 R52.1
N$76: C53.1 R52.2
N$77: C54.1 Q5.C R50.2 R51.1
N$78: C54.2 R53.1
N$79: IC7.1 R53.2
N$80: C55.1 IC7.2
N$81: C56.2 R47.P$3
N$82: C49.2 IC9.3 R47.P$1
N$83: C50.2 C65.1 C76.1 C77.1 C78.1 C79.1 C80.1 C81.1 C82.1 C83.1 C84.1 C85.1 IC9.5
N$84: IC8.3 R42.1 R43.2 R44.2
N$85: C48.2 IC8.2 R46.P$3
N$86: C46.2 C47.2 IC7.6
N$87: C47.1 R55.2
N$88: R41.1 R46.P$1
N$89: IC10.19 R56.1 SCK1.TP
N$90: IC10.18 MISO1.TP R57.1
N$91: IC10.17 MOSI1.TP R58.1
N$92: IC10.16 R59.1
N$93: IC10.15 R60.1
N$94: IC10.14 R61.1
N$95: IC10.13 R62.1
N$96: IC10.12 R63.1
N$97: IC11.5 R56.2
N$98: IC11.4 R57.2
N$99: IC11.10 R58.2
N$100: IC11.1 R59.2
N$101: IC11.2 R60.2
N$102: IC11.3 R61.2
N$103: IC11.8 R62.2
N$104: IC11.7 R63.2
N$105: IC11.9 R77.2
N$106: IC11.6 R78.2
N$107: C58.1 IC10.5 X2.3
N$108: C59.2 C60.1 IC10.20 IC12.3 R64.1 R68.1 VCC1.TP
N$109: C62.1 R64.2 R65.1 R66.1
N$110: C63.2 Q7.B R66.2
N$111: C64.1 Q7.C R65.2
N$112: C61.1 C86.1 IC12.2@1 R67.2
N$113: IC10.1 RES1.TP
N$114: C64.2 IC10.9 R68.2 R69.1
N$115: C65.2 R70.1
N$116: C88.1 IC9.1 R70.2
N$117: C63.1 R71.2
N$118: C70.2 IC7.8 IC8.7 R44.1 R49.1 R72.1
N$119: C71.1 R67.1 R73.2
N$120: C87.2 SG4.+
N$121: C87.1 Q8.B R74.1
N$122: C88.2 R75.1
N$123: IC9.8 R75.2
N$124: R76.2 U$2.P$1
N$125: SP2.+ U$2.P$5 U$2.P$6
N$126: C57.1 IC10.4 X2.1
N$127: IC10.6 R78.1
N$128: IC10.7 R77.1
N$129: C89.1 C90.1 D2.A S2.3
N$130: G2.+ S2.2
N$131: C121.2 C122.2 C123.2 C124.2 C125.2 C126.2 C127.2 C128.2 C129.2 C130.2 U$3.P$3 U$3.P$4
N$132: C95.1 R84.1
N$133: C96.2 IC15.7
N$134: IC13.4 R93.1
N$135: C101.1 R93.2
N$136: C97.2 SG5.+
N$137: C97.1 Q10.B R79.1
N$138: C98.2 Q10.C Q12.C R79.2 R87.2 R113.2
N$139: C111.1 C112.1 C113.1 C114.1 R87.1 R88.2 R89.1
N$140: Q9.B R90.2 R91.1
N$141: C98.1 R91.2
N$142: C99.1 Q9.C R89.2 R90.1
N$143: C99.2 R92.1
N$144: IC13.1 R92.2
N$145: C100.1 IC13.2
N$146: C101.2 R86.P$3
N$147: C94.2 IC15.3 R86.P$1
N$148: C95.2 C110.1 C121.1 C122.1 C123.1 C124.1 C125.1 C126.1 C127.1 C128.1 C129.1 C130.1 IC15.5
N$149: IC14.3 R81.1 R82.2 R83.2
N$150: C93.2 IC14.2 R85.P$3
N$151: C91.2 C92.2 IC13.6
N$152: C92.1 R94.2
N$153: R80.1 R85.P$1
N$154: IC16.19 R95.1 SCK2.TP
N$155: IC16.18 MISO2.TP R96.1
N$156: IC16.17 MOSI2.TP R97.1
N$157: IC16.16 R98.1
N$158: IC16.15 R99.1
N$159: IC16.14 R100.1
N$160: IC16.13 R101.1
N$161: IC16.12 R102.1
N$162: IC17.5 R95.2
N$163: IC17.4 R96.2
N$164: IC17.10 R97.2
N$165: IC17.1 R98.2
N$166: IC17.2 R99.2
N$167: IC17.3 R100.2
N$168: IC17.8 R101.2
N$169: IC17.7 R102.2
N$170: IC17.9 R116.2
N$171: IC17.6 R117.2
N$172: C103.1 IC16.5 X3.3
N$173: C104.2 C105.1 IC16.20 IC18.3 R103.1 R107.1 VCC2.TP
N$174: C107.1 R103.2 R104.1 R105.1
N$175: C108.2 Q11.B R105.2
N$176: C109.1 Q11.C R104.2
N$177: C106.1 C131.1 IC18.2@1 R106.2
N$178: IC16.1 RES2.TP
N$179: C109.2 IC16.9 R107.2 R108.1
N$180: C110.2 R109.1
N$181: C133.1 IC15.1 R109.2
N$182: C108.1 R110.2
N$183: C115.2 IC13.8 IC14.7 R83.1 R88.1 R111.1
N$184: C116.1 R106.1 R112.2
N$185: C132.2 SG6.+
N$186: C132.1 Q12.B R113.1
N$187: C133.2 R114.1
N$188: IC15.8 R114.2
N$189: R115.2 U$3.P$1
N$190: SP3.+ U$3.P$5 U$3.P$6
N$191: C102.1 IC16.4 X3.1
N$192: IC16.6 R117.1
N$193: IC16.7 R116.1
N$194: C134.1 C135.1 D3.A S3.3
N$195: G3.+ S3.2
N$196: C166.2 C167.2 C168.2 C169.2 C170.2 C171.2 C172.2 C173.2 C174.2 C175.2 U$4.P$3 U$4.P$4
N$197: C140.1 R123.1
N$198: C141.2 IC21.7
N$199: IC19.4 R132.1
N$200: C146.1 R132.2
N$201: C142.2 SG7.+
N$202: C142.1 Q14.B R118.1
N$203: C143.2 Q14.C Q16.C R118.2 R126.2 R152.2
N$204: C156.1 C157.1 C158.1 C159.1 R126.1 R127.2 R128.1
N$205: Q13.B R129.2 R130.1
N$206: C143.1 R130.2
N$207: C144.1 Q13.C R128.2 R129.1
N$208: C144.2 R131.1
N$209: IC19.1 R131.2
N$210: C145.1 IC19.2
N$211: C146.2 R125.P$3
N$212: C139.2 IC21.3 R125.P$1
N$213: C140.2 C155.1 C166.1 C167.1 C168.1 C169.1 C170.1 C171.1 C172.1 C173.1 C174.1 C175.1 IC21.5
N$214: IC20.3 R120.1 R121.2 R122.2
N$215: C138.2 IC20.2 R124.P$3
N$216: C136.2 C137.2 IC19.6
N$217: C137.1 R133.2
N$218: R119.1 R124.P$1
N$219: IC22.19 R134.1 SCK3.TP
N$220: IC22.18 MISO3.TP R135.1
N$221: IC22.17 MOSI3.TP R136.1
N$222: IC22.16 R137.1
N$223: IC22.15 R138.1
N$224: IC22.14 R139.1
N$225: IC22.13 R140.1
N$226: IC22.12 R141.1
N$227: IC23.5 R134.2
N$228: IC23.4 R135.2
N$229: IC23.10 R136.2
N$230: IC23.1 R137.2
N$231: IC23.2 R138.2
N$232: IC23.3 R139.2
N$233: IC23.8 R140.2
N$234: IC23.7 R141.2
N$235: IC23.9 R155.2
N$236: IC23.6 R156.2
N$237: C148.1 IC22.5 X4.3
N$238: C149.2 C150.1 IC22.20 IC24.3 R142.1 R146.1 VCC3.TP
N$239: C152.1 R142.2 R143.1 R144.1
N$240: C153.2 Q15.B R144.2
N$241: C154.1 Q15.C R143.2
N$242: C151.1 C176.1 IC24.2@1 R145.2
N$243: IC22.1 RES3.TP
N$244: C154.2 IC22.9 R146.2 R147.1
N$245: C155.2 R148.1
N$246: C178.1 IC21.1 R148.2
N$247: C153.1 R149.2
N$248: C160.2 IC19.8 IC20.7 R122.1 R127.1 R150.1
N$249: C161.1 R145.1 R151.2
N$250: C177.2 SG8.+
N$251: C177.1 Q16.B R152.1
N$252: C178.2 R153.1
N$253: IC21.8 R153.2
N$254: R154.2 U$4.P$1
N$255: SP4.+ U$4.P$5 U$4.P$6
N$256: C147.1 IC22.4 X4.1
N$257: IC22.6 R156.1
N$258: IC22.7 R155.1
N$259: C179.1 C180.1 D4.A S4.3
N$260: G4.+ S4.2
N$261: C211.2 C212.2 C213.2 C214.2 C215.2 C216.2 C217.2 C218.2 C219.2 C220.2 U$5.P$3 U$5.P$4
N$262: C185.1 R162.1
N$263: C186.2 IC27.7
N$264: IC25.4 R171.1
N$265: C191.1 R171.2
N$266: C187.2 SG9.+
N$267: C187.1 Q18.B R157.1
N$268: C188.2 Q18.C Q20.C R157.2 R165.2 R191.2
N$269: C201.1 C202.1 C203.1 C204.1 R165.1 R166.2 R167.1
N$270: Q17.B R168.2 R169.1
N$271: C188.1 R169.2
N$272: C189.1 Q17.C R167.2 R168.1
N$273: C189.2 R170.1
N$274: IC25.1 R170.2
N$275: C190.1 IC25.2
N$276: C191.2 R164.P$3
N$277: C184.2 IC27.3 R164.P$1
N$278: C185.2 C200.1 C211.1 C212.1 C213.1 C214.1 C215.1 C216.1 C217.1 C218.1 C219.1 C220.1 IC27.5
N$279: IC26.3 R159.1 R160.2 R161.2
N$280: C183.2 IC26.2 R163.P$3
N$281: C181.2 C182.2 IC25.6
N$282: C182.1 R172.2
N$283: R158.1 R163.P$1
N$284: IC28.19 R173.1 SCK4.TP
N$285: IC28.18 MISO4.TP R174.1
N$286: IC28.17 MOSI4.TP R175.1
N$287: IC28.16 R176.1
N$288: IC28.15 R177.1
N$289: IC28.14 R178.1
N$290: IC28.13 R179.1
N$291: IC28.12 R180.1
N$292: IC29.5 R173.2
N$293: IC29.4 R174.2
N$294: IC29.10 R175.2
N$295: IC29.1 R176.2
N$296: IC29.2 R177.2
N$297: IC29.3 R178.2
N$298: IC29.8 R179.2
N$299: IC29.7 R180.2
N$300: IC29.9 R194.2
N$301: IC29.6 R195.2
N$302: C193.1 IC28.5 X5.3
N$303: C194.2 C195.1 IC28.20 IC30.3 R181.1 R185.1 VCC4.TP
N$304: C197.1 R181.2 R182.1 R183.1
N$305: C198.2 Q19.B R183.2
N$306: C199.1 Q19.C R182.2
N$307: C196.1 C221.1 IC30.2@1 R184.2
N$308: IC28.1 RES4.TP
N$309: C199.2 IC28.9 R185.2 R186.1
N$310: C200.2 R187.1
N$311: C223.1 IC27.1 R187.2
N$312: C198.1 R188.2
N$313: C205.2 IC25.8 IC26.7 R161.1 R166.1 R189.1
N$314: C206.1 R184.1 R190.2
N$315: C222.2 SG10.+
N$316: C222.1 Q20.B R191.1
N$317: C223.2 R192.1
N$318: IC27.8 R192.2
N$319: R193.2 U$5.P$1
N$320: SP5.+ U$5.P$5 U$5.P$6
N$321: C192.1 IC28.4 X5.1
N$322: IC28.6 R195.1
N$323: IC28.7 R194.1
N$324: C224.1 C225.1 D5.A S5.3
N$325: G5.+ S5.2
N$326: C256.2 C257.2 C258.2 C259.2 C260.2 C261.2 C262.2 C263.2 C264.2 C265.2 U$6.P$3 U$6.P$4
N$327: C230.1 R201.1
N$328: C231.2 IC33.7
N$329: IC31.4 R210.1
N$330: C236.1 R210.2
N$331: C232.2 SG11.+
N$332: C232.1 Q22.B R196.1
N$333: C233.2 Q22.C Q24.C R196.2 R204.2 R230.2
N$334: C246.1 C247.1 C248.1 C249.1 R204.1 R205.2 R206.1
N$335: Q21.B R207.2 R208.1
N$336: C233.1 R208.2
N$337: C234.1 Q21.C R206.2 R207.1
N$338: C234.2 R209.1
N$339: IC31.1 R209.2
N$340: C235.1 IC31.2
N$341: C236.2 R203.P$3
N$342: C229.2 IC33.3 R203.P$1
N$343: C230.2 C245.1 C256.1 C257.1 C258.1 C259.1 C260.1 C261.1 C262.1 C263.1 C264.1 C265.1 IC33.5
N$344: IC32.3 R198.1 R199.2 R200.2
N$345: C228.2 IC32.2 R202.P$3
N$346: C226.2 C227.2 IC31.6
N$347: C227.1 R211.2
N$348: R197.1 R202.P$1
N$349: IC34.19 R212.1 SCK5.TP
N$350: IC34.18 MISO5.TP R213.1
N$351: IC34.17 MOSI5.TP R214.1
N$352: IC34.16 R215.1
N$353: IC34.15 R216.1
N$354: IC34.14 R217.1
N$355: IC34.13 R218.1
N$356: IC34.12 R219.1
N$357: IC35.5 R212.2
N$358: IC35.4 R213.2
N$359: IC35.10 R214.2
N$360: IC35.1 R215.2
N$361: IC35.2 R216.2
N$362: IC35.3 R217.2
N$363: IC35.8 R218.2
N$364: IC35.7 R219.2
N$365: IC35.9 R233.2
N$366: IC35.6 R234.2
N$367: C238.1 IC34.5 X6.3
N$368: C239.2 C240.1 IC34.20 IC36.3 R220.1 R224.1 VCC5.TP
N$369: C242.1 R220.2 R221.1 R222.1
N$370: C243.2 Q23.B R222.2
N$371: C244.1 Q23.C R221.2
N$372: C241.1 C266.1 IC36.2@1 R223.2
N$373: IC34.1 RES5.TP
N$374: C244.2 IC34.9 R224.2 R225.1
N$375: C245.2 R226.1
N$376: C268.1 IC33.1 R226.2
N$377: C243.1 R227.2
N$378: C250.2 IC31.8 IC32.7 R200.1 R205.1 R228.1
N$379: C251.1 R223.1 R229.2
N$380: C267.2 SG12.+
N$381: C267.1 Q24.B R230.1
N$382: C268.2 R231.1
N$383: IC33.8 R231.2
N$384: R232.2 U$6.P$1
N$385: SP6.+ U$6.P$5 U$6.P$6
N$386: C237.1 IC34.4 X6.1
N$387: IC34.6 R234.1
N$388: IC34.7 R233.1
N$389: C269.1 C270.1 D6.A S6.3
N$390: G6.+ S6.2

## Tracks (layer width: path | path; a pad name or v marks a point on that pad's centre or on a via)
+9V  (1 unrouted)
  Top 0.406: R35.1 51.75,48.58 | 51.75,48.58 52.07,48.26 52.07,44.2 | C1.1 52.07,40.96 52.07,43.81 52.07,44.2 | C1.1 C29.1 | IC3.6 42.55,20.95 45.09,20.95 48.9,24.77 48.9,25.72 R34.2 49.85,26.04 50.48,26.67 50.48,27.94 50.48,31.43 C31.1 C30.1 C1.1 | 50.16,38.73 52.7,38.73 | 51.75,48.58 | D1.C 52.07,44.2
+9V1  (1 unrouted)
  Top 0.406: R73.1 120.33,48.58 | 120.33,48.58 120.65,48.26 120.65,44.2 | C72.1 120.65,40.96 120.65,43.81 120.65,44.2 | C72.1 C73.1 | IC9.6 111.12,20.95 113.67,20.95 117.47,24.77 117.47,25.72 R72.2 118.43,26.04 119.06,26.67 119.06,27.94 119.06,31.43 C75.1 C74.1 C72.1 | 118.75,38.73 121.28,38.73 | 120.33,48.58 | D2.C 120.65,44.2
+9V2  (1 unrouted)
  Top 0.406: R112.1 188.91,48.58 | 188.91,48.58 189.23,48.26 189.23,44.2 | C117.1 189.23,40.96 189.23,43.81 189.23,44.2 | C117.1 C118.1 | IC15.6 179.71,20.95 182.25,20.95 186.06,24.77 186.06,25.72 R111.2 187.01,26.04 187.64,26.67 187.64,27.94 187.65,31.43 C120.1 C119.1 C117.1 | 187.32,38.73 189.87,38.73 | 188.91,48.58 | D3.C 189.23,44.2
+9V3  (1 unrouted)
  Top 0.406: R151.1 51.75,109.54 | 51.75,109.54 52.07,109.22 52.07,105.17 | C162.1 52.07,101.92 52.07,104.78 52.07,105.17 | C162.1 C163.1 | IC21.6 42.55,81.92 45.09,81.92 48.9,85.72 48.9,86.68 R150.2 49.85,87 50.48,87.63 50.48,88.9 50.48,92.39 C165.1 C164.1 C162.1 | 50.16,99.69 52.7,99.69 | 51.75,109.54 | D4.C 52.07,105.17
+9V4  (1 unrouted)
  Top 0.406: R190.1 120.33,109.54 | 120.33,109.54 120.65,109.22 120.65,105.17 | C207.1 120.65,101.92 120.65,104.78 120.65,105.17 | C207.1 C208.1 | IC27.6 111.12,81.92 113.67,81.92 117.47,85.72 117.47,86.68 R189.2 118.43,87 119.06,87.63 119.06,88.9 119.06,92.39 C210.1 C209.1 C207.1 | 118.75,99.69 121.28,99.69 | 120.33,109.54 | D5.C 120.65,105.17
+9V5  (1 unrouted)
  Top 0.406: R229.1 188.91,109.54 | 188.91,109.54 189.23,109.22 189.23,105.17 | C252.1 189.23,101.92 189.23,104.78 189.23,105.17 | C252.1 C253.1 | IC33.6 179.71,81.92 182.25,81.92 186.06,85.72 186.06,86.68 R228.2 187.01,87 187.64,87.63 187.64,88.9 187.65,92.39 C255.1 C254.1 C252.1 | 187.32,99.69 189.87,99.69 | 188.91,109.54 | D6.C 189.23,105.17
-1V  (via drill 0.5)
  Top 0.406: R11.2 36.83,21.59 | 36.83,21.59 35.56,22.86 34.92,22.86 34.29,23.5 28.57,23.5 27.94,22.86 IC2.6 | 36.83,21.59 v36.83,22.23 38.42,22.23 39.05,22.86 39.05,24.13 | v33.34,15.88 R10.2 | 40.05,26.3 R9.1 39.69,26.36 39.05,25.72 39.05,24.13 | R33.1 39.37,24.45 39.05,24.13
  Bottom 0.406: v36.83,22.23 36.83,19.37 v33.34,15.88
-1V1  (via drill 0.5)
  Top 0.406: R42.2 105.41,21.59 | 105.41,21.59 104.14,22.86 103.5,22.86 102.87,23.5 97.16,23.5 96.52,22.86 IC8.6 | 105.41,21.59 v105.41,22.23 107,22.23 107.63,22.86 107.63,24.13 | v101.92,15.88 R41.2 | 108.64,26.3 R55.1 108.27,26.36 107.63,25.72 107.63,24.13 | R71.1 107.95,24.45 107.63,24.13
  Bottom 0.406: v105.41,22.23 105.41,19.37 v101.92,15.88
-1V2  (via drill 0.5)
  Top 0.406: R81.2 173.99,21.59 | 173.99,21.59 172.72,22.86 172.09,22.86 171.45,23.5 165.74,23.5 165.1,22.86 IC14.6 | 173.99,21.59 v173.99,22.23 175.58,22.23 176.21,22.86 176.21,24.13 | v170.5,15.88 R80.2 | 177.22,26.3 R94.1 176.85,26.36 176.21,25.72 176.21,24.13 | R110.1 176.53,24.45 176.21,24.13
  Bottom 0.406: v173.99,22.23 173.99,19.37 v170.5,15.88
-1V3  (via drill 0.5)
  Top 0.406: R120.2 36.83,82.55 | 36.83,82.55 35.56,83.82 34.92,83.82 34.29,84.45 28.57,84.45 27.94,83.82 IC20.6 | 36.83,82.55 v36.83,83.19 38.42,83.19 39.05,83.82 39.05,85.09 | v33.34,76.83 R119.2 | 40.05,87.27 R133.1 39.69,87.31 39.05,86.68 39.05,85.09 | R149.1 39.37,85.41 39.05,85.09
  Bottom 0.406: v36.83,83.19 36.83,80.33 v33.34,76.83
-1V4  (via drill 0.5)
  Top 0.406: R159.2 105.41,82.55 | 105.41,82.55 104.14,83.82 103.5,83.82 102.87,84.45 97.16,84.45 96.52,83.82 IC26.6 | 105.41,82.55 v105.41,83.19 107,83.19 107.63,83.82 107.63,85.09 | v101.92,76.83 R158.2 | 108.64,87.27 R172.1 108.27,87.31 107.63,86.68 107.63,85.09 | R188.1 107.95,85.41 107.63,85.09
  Bottom 0.406: v105.41,83.19 105.41,80.33 v101.92,76.83
-1V5  (via drill 0.5)
  Top 0.406: R198.2 173.99,82.55 | 173.99,82.55 172.72,83.82 172.09,83.82 171.45,84.45 165.74,84.45 165.1,83.82 IC32.6 | 173.99,82.55 v173.99,83.19 175.58,83.19 176.21,83.82 176.21,85.09 | v170.5,76.83 R197.2 | 177.22,87.27 R211.1 176.85,87.31 176.21,86.68 176.21,85.09 | R227.1 176.53,85.41 176.21,85.09
  Bottom 0.406: v173.99,83.19 173.99,80.33 v170.5,76.83
GND  (via drill 0.5)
